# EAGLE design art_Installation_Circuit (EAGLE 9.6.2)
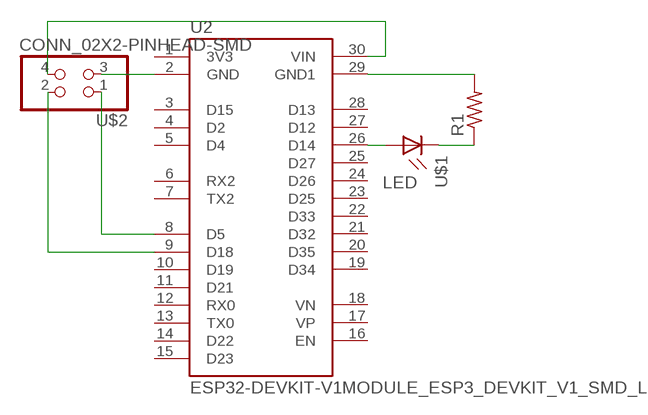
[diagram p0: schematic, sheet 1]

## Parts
R1  R1206  [R1206]
U2  ESP32-DEVKIT-V1MODULE_ESP3_DEVKIT_V1_SMD_LONG  [MODULE_ESP32_DEVKIT_V1_SMD_LONG]
U$1  LED  [LED1206]
U$2  CONN_02X2-PINHEAD-SMD  [2X02SMD]

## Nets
N$1: U2.2(GND) U$2.3
N$2: U2.8(D5) U$2.1
N$3: U2.30(VIN) U$2.4
N$4: U2.9(D18) U$2.2
N$5: R1.2 U2.29(GND1)
N$6: U2.26(D14) U$1.1(A)
N$7: R1.1 U$1.2(C)
Unconnected: U2.1(3V3) U2.3(D15) U2.4(D2) U2.5(D4) U2.6(RX2) U2.7(TX2) U2.10(D19) U2.11(D21) U2.12(RX0) U2.13(TX0) U2.14(D22) U2.15(D23) U2.16(EN) U2.17(VP) U2.18(VN) U2.19(D34) U2.20(D35) U2.21(D32) U2.22(D33) U2.23(D25) U2.24(D26) U2.25(D27) U2.27(D12) U2.28(D13)

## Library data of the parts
R1 = fab-emma-re8nowiwt7yj8fhybscymuq61o:R: Resistor (US Symbol)
U2 = ESP32-DEVKIT-V1:ESP32-DEVKIT-V1: Dual core, Wi-Fi: 2.4 GHz up to 150 Mbits/s,BLE (Bluetooth Low Energy) and legacy Bluetooth, 32 bits, Up to 240 MHz Check availability
U$1 = fab-emma-re8nowiwt7yj8fhybscymuq61o:LED: LED
U$2 = fab-emma-re8nowiwt7yj8fhybscymuq61o:CONN_02X2-PINHEAD-SMD

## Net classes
0 default: width 0.4 mm, clearance 0.4 mm

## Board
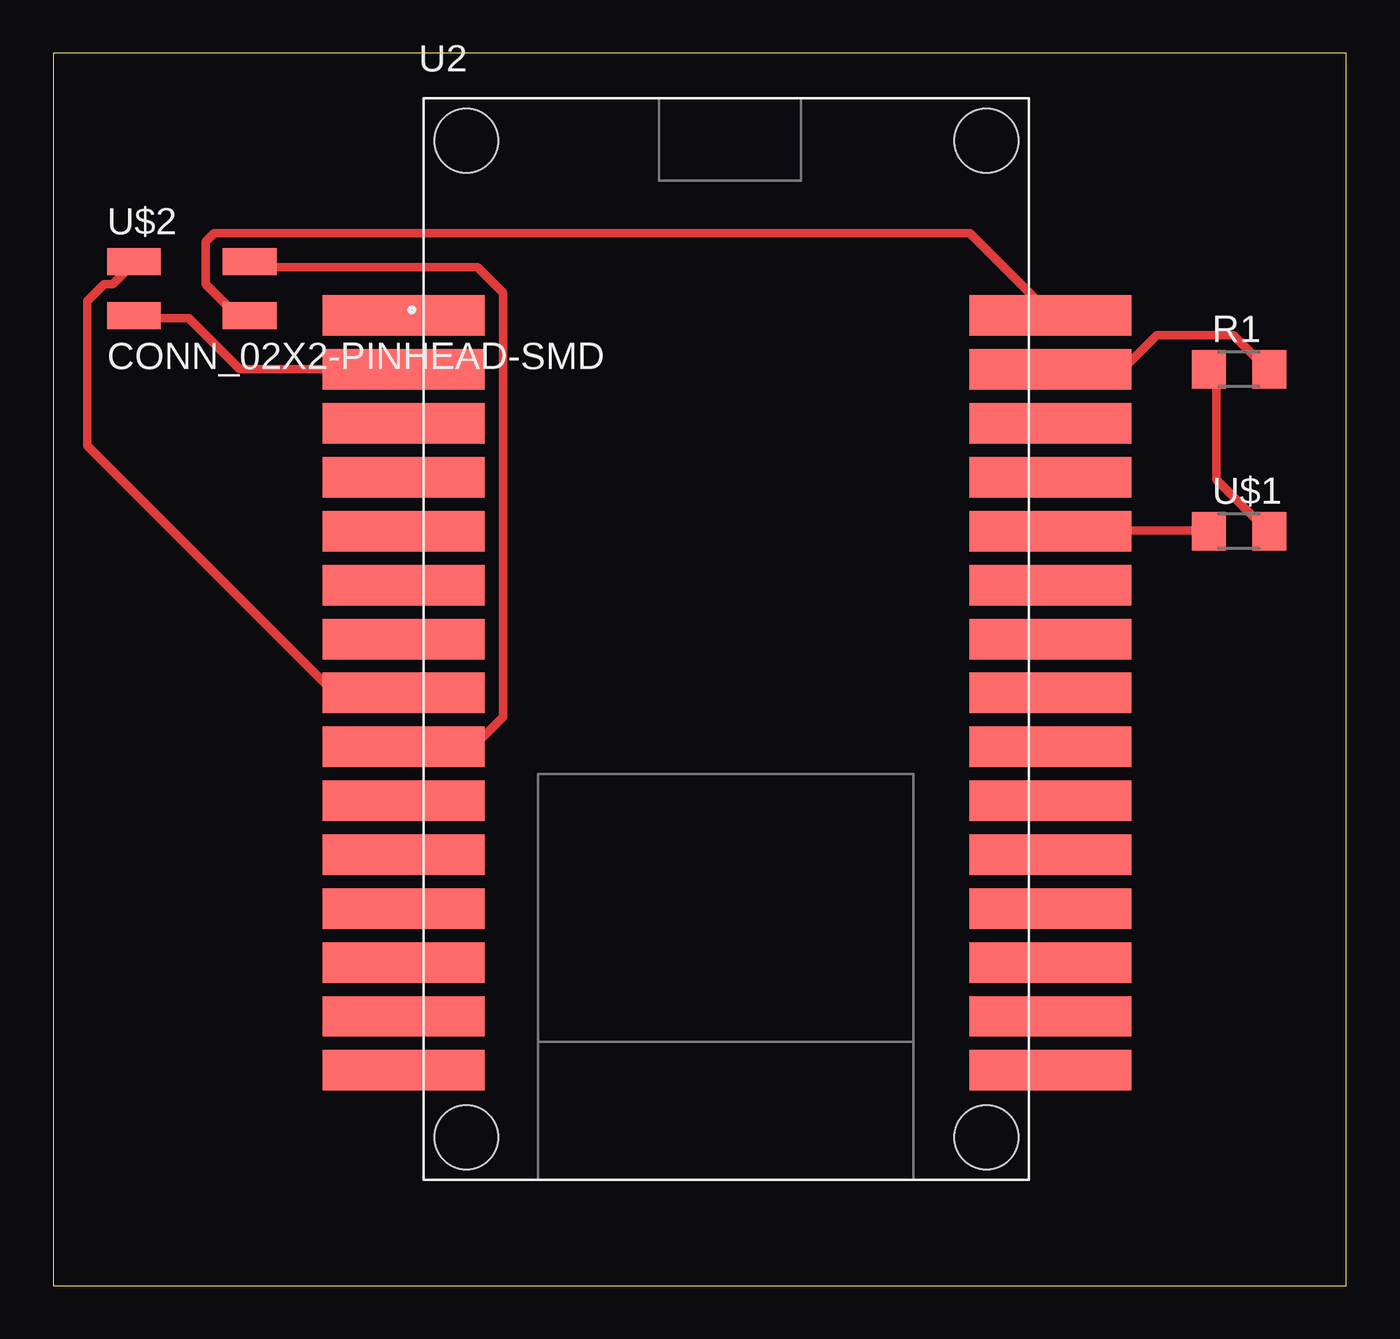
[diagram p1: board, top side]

Size 60.94 x 58.09 mm. Coordinates in mm from the lower left corner, seen from the top.
Outline: 0,0 60.94,0 60.94,58.09 0,58.09 0,0
Copper layers (1*16): Top 0.035mm / dielectric 1.5mm / Bottom 0.035mm
Design rules "default *": minimum track width 6mil, minimum drill 0.35mm, track to track 0.4mm, track to pad 0.4mm, pad to pad 0.4mm, via to via 0.4mm, smd to smd 0.4mm, copper to edge 0.4mm, drill to drill 6mil, minimum pad ring 10mil, minimum via ring 8mil, stop-mask expansion 4mil, vias tented up to drill 0mil, thermal gap 10mil

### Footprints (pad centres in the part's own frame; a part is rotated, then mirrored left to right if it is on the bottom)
R1206 = smd 1.6 x 1.803: 1 -1.422,0; 2 1.422,0
MODULE_ESP32_DEVKIT_V1_SMD_LONG = smd 7.62 x 1.905: 1 -15.24,15.24; 2 -15.24,12.7; 3 -15.24,10.16; 4 -15.24,7.62; 5 -15.24,5.08; 6 -15.24,2.54; 7 -15.24,0; 8 -15.24,-2.54; 9 -15.24,-5.08; 10 -15.24,-7.62; 11 -15.24,-10.16; 12 -15.24,-12.7; 13 -15.24,-15.24; 14 -15.24,-17.78; 15 -15.24,-20.32; 16 15.24,-20.32; 17 15.24,-17.78; 18 15.24,-15.24; 19 15.24,-12.7; 20 15.24,-10.16; 21 15.24,-7.62; 22 15.24,-5.08; 23 15.24,-2.54; 24 15.24,0; 25 15.24,2.54; 26 15.24,5.08; 27 15.24,7.62; 28 15.24,10.16; 29 15.24,12.7; 30 15.24,15.24 | hole 3: -12.28,-23.475; 12.23,-23.475; 12.23,23.475; -12.28,23.475
LED1206 = smd 1.6 x 1.803: 1 -1.422,0; 2 1.422,0
2X02SMD = smd 2.54 x 1.27: 1 -2.54,1.27; 2 2.92,1.27; 3 -2.54,-1.27; 4 2.92,-1.27

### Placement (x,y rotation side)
R1  55.88,43.18 0 top
U2  31.75,30.48 0 top
U$1  55.88,35.56 0 top
U$2  6.35,46.99 0 top

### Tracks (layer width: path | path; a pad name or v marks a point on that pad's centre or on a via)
N$1
  Top 0.4: U$2.3 4,45.6 6.4,45.6 8.8,43.2 16.4,43.2 U2.2
N$2
  Top 0.4: U$2.1 3.6,48 2.8,47.2 2.4,47.2 1.6,46.4 1.6,39.6 13.2,28 16.4,28 U2.8
N$3
  Top 0.4: U$2.4 9.2,46 8.4,46 7.2,47.2 7.2,49.2 7.6,49.6 43.2,49.6 46.8,46 U2.30
N$4
  Top 0.4: U$2.2 9.6,48 20,48 21.2,46.8 21.2,26.8 20,25.6 16.8,25.6 U2.9
N$5
  Top 0.4: R1.2 57.2,43.2 55.6,44.8 52,44.8 50.4,43.2 47.2,43.2 U2.29
N$6
  Top 0.4: U$1.1 54.4,35.6 47.2,35.6 U2.26
N$7
  Top 0.4: R1.1 54.8,42.8 54.8,38 57.2,35.6 U$1.2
